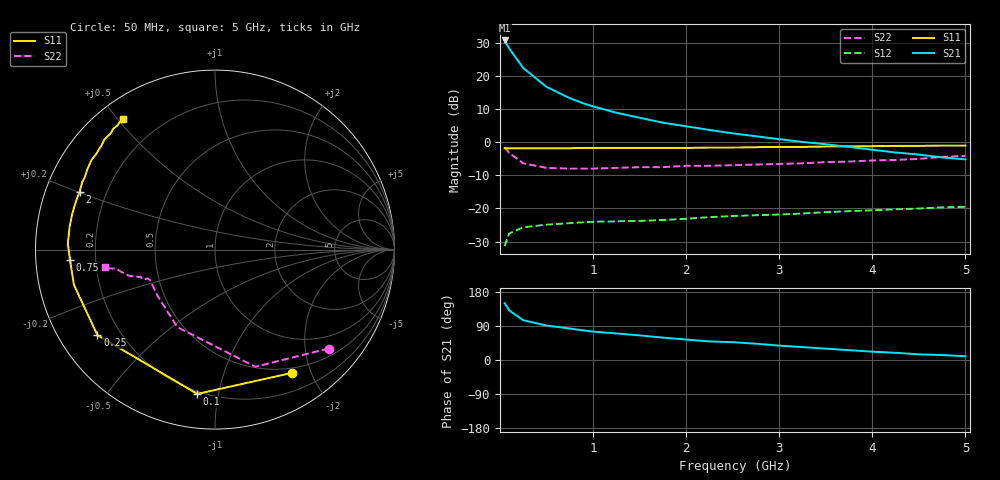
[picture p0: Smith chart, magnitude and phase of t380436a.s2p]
!AT-38043
!S-PARAMETERS at Vce=6.0V Ic=50mA. LAST UPDATED 01-06-98
# ghz s ma r 50
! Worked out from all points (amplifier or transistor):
!   23 points, 50 MHz to 5 GHz, reference 50 ohm
!   highest |S21| = 30.7 dB at 50 MHz (marker M1)
!   |S21| within 3 dB of that: start of sweep to 115.2 MHz
!   unconditionally stable (mu >= 1): 1.63 GHz to end of sweep
!   at 500 MHz: K = 0.39, MSG = 20.8 dB, |S12| = -24.9 dB
!   at 2.25 GHz: K = 1.18, MAG = 10.6 dB, |S12| = -22.6 dB
!   at 5 GHz: K = 1.24, MAG = 4.2 dB, |S12| = -19.5 dB
!   S11 on the Smith chart (normalised r, x): 50 MHz: 0.43, -1.72; 100 MHz: 0.19, -0.87; 250 MHz: 0.12, -0.32; 750 MHz: 0.11, -0.03; 2 GHz: 0.10, +0.20; 5 GHz: 0.07, +0.52
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0.05  0.81 -58.0  34.28 150.0  0.027 58.0  0.84 -41.0
0.1  0.81 -97.0  26 131.0  0.042 45.0  0.69 -71.0
0.25  0.81 -144.0  13.18 105.0  0.052 25.0  0.48 -116.0
0.5  0.81 -166.0  6.84 91.0  0.057 20.0  0.41 -142.0
0.75  0.81 -176.0  4.62 83.0  0.06 21.0  0.4 -151.0
0.9  0.82 178.0  3.85 78.0  0.062 21.0  0.4 -154.0
1  0.82 177.0  3.47 75.0  0.063 23.0  0.4 -155.0
1.25  0.82 171.0  2.79 70.0  0.064 24.0  0.41 -157.0
1.5  0.82 166.0  2.34 65.0  0.065 28.0  0.42 -157.0
1.75  0.82 161.0  1.97 59.0  0.067 31.0  0.42 -158.0
2  0.82 157.0  1.74 54.0  0.07 33.0  0.44 -159.0
2.25  0.83 153.0  1.53 49.0  0.074 36.0  0.44 -160.0
2.5  0.83 151.0  1.36 47.0  0.077 39.0  0.45 -160.0
2.75  0.84 148.0  1.23 43.0  0.079 43.0  0.46 -161.0
3  0.85 144.0  1.11 38.0  0.081 44.0  0.47 -162.0
3.5  0.86 137.0  0.93 30.0  0.088 45.0  0.5 -163.0
3.75  0.87 135.0  0.85 26.0  0.091 45.0  0.51 -164.0
4  0.87 132.0  0.77 22.0  0.094 45.0  0.53 -166.0
4.25  0.88 130.0  0.7 19.0  0.097 46.0  0.54 -167.0
4.5  0.88 128.0  0.65 15.0  0.1 46.0  0.56 -169.0
4.75  0.89 126.0  0.59 13.0  0.104 46.0  0.6 -170.0
5  0.89 125.0  0.55 10.0  0.106 46.0  0.62 -171.0
